FUNCTION_BLOCK TL_CNC_Axis
VAR_INPUT
	TorquePermission	: BOOL;
	ReleaseFeedhold		: BOOL;
	CommunicationReady	: BOOL;
	/// AxisTracking = true means, CNC should set commanded position to actual position 
	AxisTracking		: BOOL;
	HomingDone			: BOOL;
	inc_per_unit	: LREAL := 1E7; (* use 10000 inc/deg or 1E7 inc/m *)
END_VAR
VAR_OUTPUT
	CNC_Referenced		: BOOL;
	messageHandler		: TL_AxisMessageHandler;
END_VAR
VAR
	/// CNC > GEO > Axis > Inputs > Sercos Phase
	SercosPhase AT %Q*	: WORD;
	/// CNC > GEO > Axis > Inputs > Drive status word
	SercosStatus AT %Q*	: WORD;
	/// CNC > GEO > Axis > Outputs > Position command value 
	SercosPosCmd AT %I*	: DINT;
	/// CNC > GEO > Axis > Inputs > Position feedback 1 value
	SercosPosAct AT %Q*	: DINT;
	
	pAxis: POINTER TO High_Level_Interface_Ax;
	
	twincatEventLib		: TL_TwinCatError;  // Events of the library-axis
	twincatEventDrv		: TL_TwinCatError;  // Events of a drive axis
END_VAR

(* --------------------------------------------- *)
(* Triamec Motion AG, 6340 Baar, Switzerland     *)
(* Sample Code may be adapted to customer need   *)
(* --------------------------------------------- *)

(* 
	we do not want any offset beween drive and cnc 
    because the drives have there own setPosition
	therefore set the following parameters in the axis of the cnc:
		kenngr.abs_pos_gueltig			1
		kenngr.set_refpos_mode         	OFFSET
		kenngr.set_refpos_offset		0
	this mode ensures, that the cnc does not set cmdPos=actPos when
	MCControlBoolUnit_SetReferencePosition is set
 
*)
;

METHOD CallFastPosAct
VAR_INPUT
	iPositionAct		: LREAL;
END_VAR

(* coerse position to DINT range *)
IF ABS(iPositionAct * inc_per_unit) < 16#7FFFFFFF  THEN
	SercosPosAct := DINT_TO_DWORD(LREAL_TO_DINT(iPositionAct * inc_per_unit));
ELSIF iPositionAct < 0 THEN
	SercosPosAct := 16#80000000;
ELSE
	SercosPosAct := 16#7FFFFFFF;
END_IF
END_METHOD

METHOD CallFastPosCmd : LREAL
VAR_INPUT
END_VAR
CallFastPosCmd := DINT_TO_LREAL( SercosPosCmd ) / inc_per_unit;
END_METHOD

METHOD CallSlow
VAR_IN_OUT
	axis				: TL_MC_AXIS_REF;
END_VAR
(* ========================================================= *)
(*    FUN: HLI_SetAxisFeedHold                               *)
(* --------------------------------------------------------- *)
(*   Author-origin: MK                                       *)
(*   Date: 10.06.2009                                        *)
(*   Rev.: 1.1                                               *)
(* ========================================================= *)
(* ========================================================= *)
(*    FUN: HLI_SetAxisTrackingOperation                      *)
(* --------------------------------------------------------- *)
(*   Author: TV                                              *)
(*   Date: 15.09.2006                                        *)
(*   Rev.: 1.0                                               *)
(* ========================================================= *)
(*   Author-mod: MVX, Triamec : added sercosePhase and Status*)

IF gHli.initialized AND axis.iAxis >= 1 AND HLI_SYS_AX_MaxIdx >= axis.iAxis THEN	(* check for axis no *)
	(* be careful, array indices start with 0 in TwinCAT 3. Axis starts with 1 *)
	pAxis	:= gpAx[axis.iAxis-1];
	pAxis^.head.plc_present_w := TRUE;

	(* enable PLC to drive HLI interface *)
	pAxis^.lr_mc_control.torque_permission.enable_w			:= TRUE;
	pAxis^.lr_mc_control.release_feedhold.enable_w 			:= TRUE;
	pAxis^.lr_mc_control.drive_on.enable_w 					:= TRUE;
	pAxis^.lr_mc_control.set_reference_position.enable_w	:= TRUE;
	pAxis^.lr_mc_control.follow_up.enable_w 				:= TRUE;

			
	(* enable external commanding of an axis *)
	(*		pAxis^.lr_mc_control.add_cmd_values.enable_w 			:= TRUE; *)
	

	(* set regulation and feed *)
	pAxis^.lr_mc_control.torque_permission.command_w		:= TorquePermission;
	pAxis^.lr_mc_control.release_feedhold.command_w 		:= ReleaseFeedhold;
	pAxis^.lr_mc_control.drive_on.command_w 				:= CommunicationReady;

	sercosPhase	:= 4 * BOOL_TO_WORD(CommunicationReady);
	sercosStatus:=   16#8000 * BOOL_TO_WORD(ReleaseFeedhold)
					+  16#4000 * BOOL_TO_WORD(TorquePermission OR (CommunicationReady AND NOT(ReleaseFeedhold)));

	(* The axis is set to tracking operation (follow up) on or off, i.e. the control loop is opened.
	   The command position implicitly is set to the actual position. *)
	pAxis^.lr_mc_control.follow_up.command_w := AxisTracking;

	(* HomingPosition *)
	pAxis^.lr_mc_control.set_reference_position.command_w	:= HomingDone;
	CNC_Referenced := pAxis^.lr_state.homing_done_r;

END_IF

// This reads the drive message string into messageHandler.messageString and then sets messageHandler.done
messageHandler.execute := axis.messageId >= TL_Message.Error; // show only errors
messageHandler(axis:=axis, Trialink:=gTrialink);

// This generates a TwinCAT event in case of an axis library error and an axis drive error
twincatEventLib.Execute	:= gTrialink.Done AND NOT (gTrialink.Error OR axis.simulate);
twincatEventLib.errorId	:= axis.errorId;
twincatEventLib.source	:= TL_EventSourceId.AxisLib; // See source entry in the ecpx file triamecEventsTrialinkLib*.ecpx
twincatEventLib.par1	:= axis.iAxis;
twincatEventLib();

twincatEventDrv.Execute	:= twincatEventLib.Execute AND axis.messageId>=TL_Message.Error; // show only errors 
twincatEventDrv.errorId	:= axis.messageId;
twincatEventDrv.source	:= TL_EventSourceId.AxisDrive; // See source entry in the ecpx file triamecEventsDrive*.ecpx
twincatEventDrv.par1	:= axis.iAxis;
twincatEventDrv();
END_METHOD

END_FUNCTION_BLOCK
